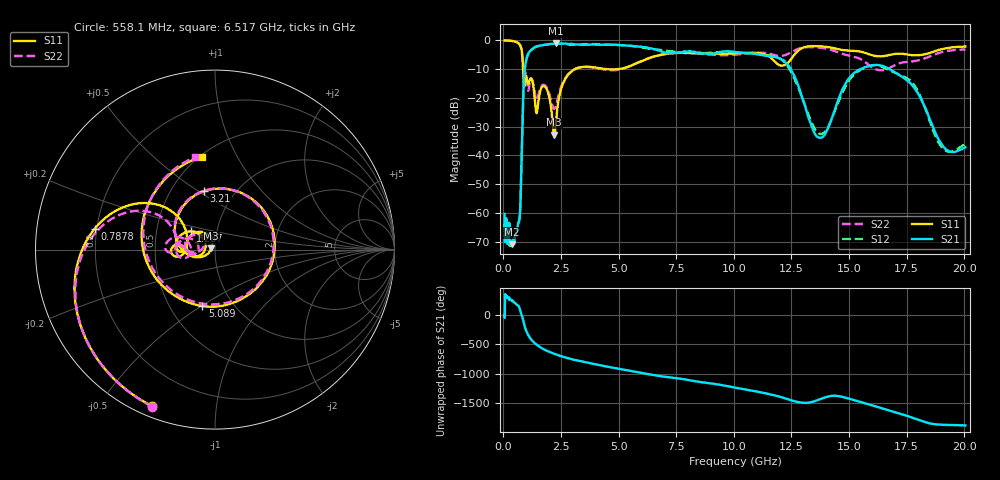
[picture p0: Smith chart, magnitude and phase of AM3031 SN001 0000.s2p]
# Hz S DB R 50
!freq MagS11 AngS11 MagS21 AngS21 MagS12 AngS12 MagS22 AngS22
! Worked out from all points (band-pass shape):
!   1601 points, 50 MHz to 20.05 GHz, reference 50 ohm
!   highest |S21| = -1.04 dB at 2.291 GHz (marker M1); lowest = -70.9 dB at 357.4 MHz (marker M2)
!   |S21| within 3 dB of the highest: 1.119 GHz to 6.919 GHz (5.8 GHz wide, 144 % of centre); 9.411 GHz to 10.08 GHz (673.5 MHz wide, 6.91 % of centre)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
!   lowest |S11| = -32.7 dB at 2.207 GHz (marker M3), VSWR 1.05, Z = 47.8 + j0.658 ohm
!   |S11| at or under -10 dB: 854.2 MHz to 3.095 GHz (2.241 GHz wide, 113 % of centre); 4.488 GHz to 4.93 GHz (441.9 MHz wide, 9.39 % of centre)
!   |S22| runs from -23.8 to 0.0 dB; largest |S21 - S12| = 0.067
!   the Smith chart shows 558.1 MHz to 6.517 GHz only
!   S11 on the Smith chart (normalised r, x): 558.1 MHz: 0.05, -0.67; 787.8 MHz: 0.19, +0.08; 1.287 GHz: 0.75, +0.16; 3.21 GHz: 0.72, +0.53; 5.089 GHz: 0.72, -0.50; 6.517 GHz: 0.51, +0.73
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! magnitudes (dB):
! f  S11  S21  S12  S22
! 50 MHz  0.0  -60.3  -64.1  0.0
! 135.9 MHz  0.0  -68.7  -68.0  0.0
! 357.4 MHz  -0.2  -70.9  -71.0  -0.2
! 369.6 MHz  -0.2  -70.6  -70.7  -0.2
! 558.1 MHz  -0.5  -66.7  -66.7  -0.5
! 709.4 MHz  -1.5  -61.2  -60.7  -1.5
! 787.8 MHz  -3.3  -40.4  -40.2  -3.5
! 881.5 MHz  -14.7  -14.6  -14.7  -13.2
! 1.005 GHz  -12.9  -6.3  -6.2  -13.2
! 1.287 GHz  -15.4  -2.8  -2.8  -14.8
! 1.872 GHz  -16.8  -1.4  -1.5  -16.3
! 2.207 GHz  -32.7  -1.1  -1.1  -23.8
! 2.291 GHz  -27.5  -1.0  -1.1  -22.2
! 2.722 GHz  -12.9  -1.1  -1.3  -12.6
! 3.21 GHz  -9.6  -1.4  -1.4  -9.6
! 5.089 GHz  -9.8  -1.6  -1.6  -10.0
! 6.517 GHz  -5.6  -3.0  -3.0  -5.6
! 7.402 GHz  -4.4  -4.3  -4.0  -4.4
! 11.91 GHz  -8.3  -6.0  -6.0  -5.3
! 13.73 GHz  -2.0  -33.8  -32.5  -2.5
! 16.44 GHz  -5.5  -8.8  -9.2  -10.4
! 20.05 GHz  -2.1  -37.1  -36.1  -3.1
